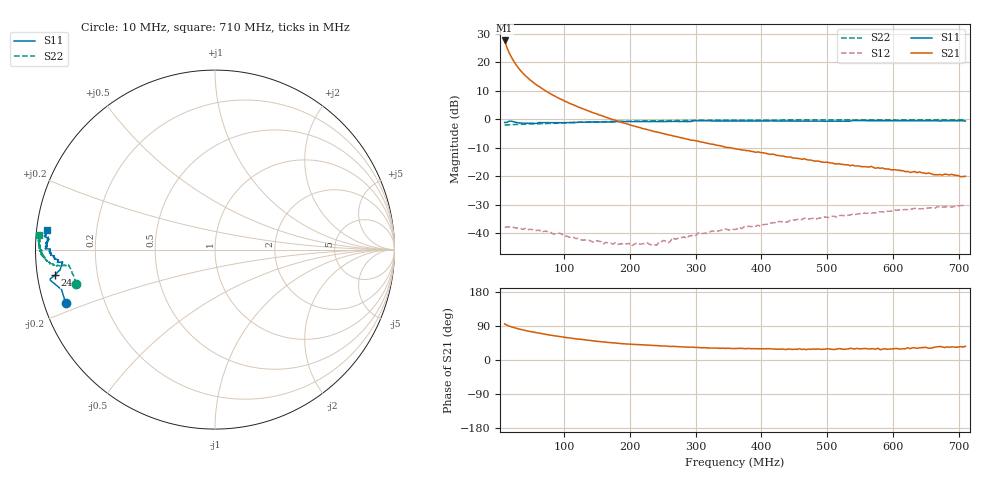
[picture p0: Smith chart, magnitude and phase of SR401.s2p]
!  POLYFET RF DEVICES
!  S PARAMETERS FOR
!  SR401 (EACH SIDE)
!  VDS=28, IDQ=600MA
! Date: Mon Jan 21 15:37:56 2002
# MHZ S MA R 50
! SCATTERING PARAMETERS :
!FREQ-MHZ MAG[S11] ANG[S11] MAG[S21] ANG[S21] MAG[S12] ANG[S12] MAG[S22] ANG[S22]
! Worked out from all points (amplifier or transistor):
!   201 points, 10 MHz to 710 MHz, reference 50 ohm
!   highest |S21| = 27.7 dB at 10 MHz (marker M1)
!   |S21| within 3 dB of that: start of sweep to 14.44 MHz
!   unconditionally stable (mu >= 1): 102.5 MHz to end of sweep
!   at 125.5 MHz: K = 1.17, MAG = 20.6 dB, |S12| = -42.3 dB
!   at 360 MHz: K = 1.34, MAG = 10.7 dB, |S12| = -38.7 dB
!   at 710 MHz: K = 1.29, MAG = 1.8 dB, |S12| = -30.0 dB
!   S11 on the Smith chart (normalised r, x): 10 MHz: 0.06, -0.17; 24 MHz: 0.05, -0.08; 710 MHz: 0.03, +0.06
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10  0.8834 -160.4  24.39 95.3  0.01261 7.1  0.7981 -166.0
13.5  0.8838 -165.4  18.3 92.0  0.01294 4.8  0.8001 -169.3
17  0.9334 -169.5  14.74 89.3  0.01287 2.9  0.807 -170.8
20.5  0.9326 -169.9  12.29 87.5  0.01281 3.7  0.8055 -171.9
24  0.9037 -170.9  10.5 85.7  0.01268 0.5  0.8122 -172.6
27.5  0.8846 -171.9  9.082 84.0  0.01229 -1.8  0.8153 -173.1
31  0.871 -172.5  8.012 82.1  0.01236 -2.2  0.8156 -173.5
34.5  0.8631 -173.6  7.14 80.8  0.01205 -2.1  0.819 -173.7
38  0.8589 -173.9  6.445 79.3  0.01165 -2.7  0.8201 -174.0
41.5  0.8581 -174.5  5.872 77.9  0.01217 -1.4  0.8213 -173.8
48.5  0.8548 -174.7  4.965 75.3  0.01174 -2.6  0.8305 -174.1
55.5  0.8561 -175.2  4.279 72.8  0.01105 -3.4  0.8374 -173.9
69.5  0.8761 -175.6  3.327 68.3  0.01079 -5.7  0.8437 -174.1
87  0.8763 -175.9  2.539 63.6  0.00969 -6.6  0.8604 -174.1
108  0.8803 -176.3  1.932 58.4  0.00851 -4.7  0.8764 -174.2
129  0.8945 -176.8  1.536 54.1  0.00754 4.1  0.8919 -174.3
174.5  0.8967 -177.7  0.9914 45.2  0.00643 15.5  0.9182 -175.0
244.5  0.9177 -179.1  0.5885 37.5  0.00699 55.9  0.9461 -176.7
360  0.9384 178.6  0.3068 30.2  0.01161 82.3  0.9703 -179.3
479  0.9338 176.7  0.1875 29.2  0.01828 88.5  0.9788 178.3
594.5  0.9479 174.5  0.133 28.9  0.02427 93.4  0.9804 176.4
710  0.9404 173.3  0.09999 36.1  0.03163 95.4  0.9849 175.4
